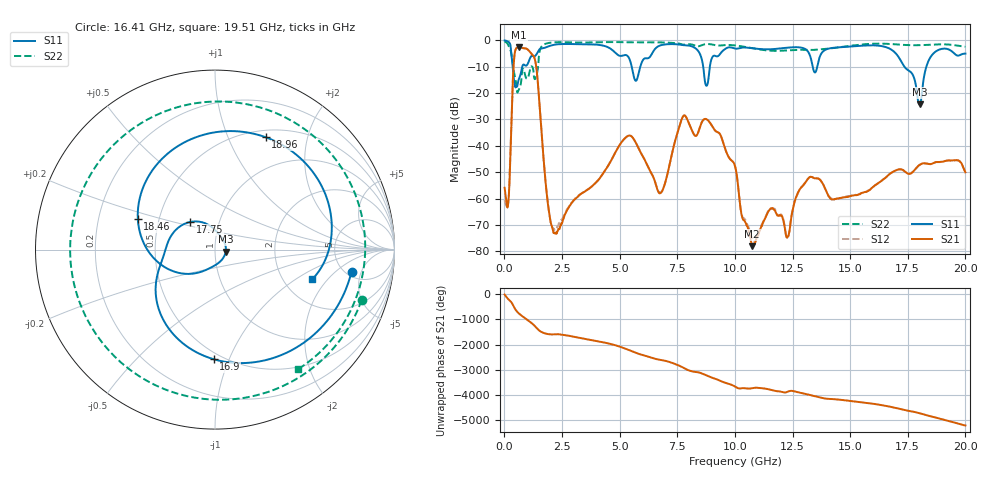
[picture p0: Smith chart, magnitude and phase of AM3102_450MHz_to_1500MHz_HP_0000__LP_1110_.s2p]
!Agilent Technologies,E8364B,MY43040894,A.07.50.67
!Agilent E8364B: A.07.50.67
!Date: Thursday, January 11, 2018 05:18:35
!Correction: S11(Full 2 Port(1,2))
!S21(Full 2 Port(1,2))
!S12(Full 2 Port(1,2))
!S22(Full 2 Port(1,2))
!S2P File: Measurements: S11, S21, S12, S22:
# Hz S  dB  R 50
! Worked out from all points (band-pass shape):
!   1601 points, 10 MHz to 20 GHz, reference 50 ohm
!   highest |S21| = -2.59 dB at 634.7 MHz (marker M1); lowest = -78.1 dB at 10.75 GHz (marker M2)
!   |S21| within 3 dB of the highest: 439 MHz to 1.232 GHz (792.8 MHz wide, 94.9 % of centre)
!   lowest |S11| = -24.3 dB at 18.01 GHz (marker M3), VSWR 1.13, Z = 56.3 - j1.3 ohm
!   |S11| at or under -10 dB: 358.5 MHz to 774.2 MHz (415.6 MHz wide, 73.4 % of centre); 5.524 GHz to 5.897 GHz (373.3 MHz wide, 6.54 % of centre); 17.36 GHz to 18.31 GHz (950.9 MHz wide, 5.33 % of centre)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
!   |S22| runs from -19.8 to -0.5 dB; largest |S21 - S12| = 0.0019
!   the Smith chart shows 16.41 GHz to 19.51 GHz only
!   S11 on the Smith chart (normalised r, x): 16.41 GHz: 5.62, -3.39; 16.9 GHz: 0.45, -0.88; 17.75 GHz: 0.73, +0.23; 18.46 GHz: 0.38, +0.16; 18.96 GHz: 0.58, +1.38; 19.51 GHz: 2.85, -1.39
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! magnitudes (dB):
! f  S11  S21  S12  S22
! 10 MHz  -0.1  -55.9  -60.7  -0.5
! 172.4 MHz  -0.6  -61.3  -61.2  -1.9
! 422.3 MHz  -15.4  -7.0  -7.0  -12.3
! 634.7 MHz  -14.6  -2.6  -2.6  -18.6
! 1.347 GHz  -5.8  -8.1  -8.1  -14.5
! 2.109 GHz  -1.8  -72.3  -71.3  -0.8
! 3.346 GHz  -1.5  -58.1  -58.1  -0.8
! 5.42 GHz  -7.0  -36.1  -36.1  -0.7
! 6.682 GHz  -2.2  -57.5  -57.3  -0.8
! 7.794 GHz  -1.8  -28.5  -28.5  -1.7
! 10.01 GHz  -3.1  -47.7  -47.6  -1.9
! 10.75 GHz  -3.0  -78.1  -74.9  -3.0
! 13.34 GHz  -8.5  -51.8  -51.9  -3.6
! 16.41 GHz  -2.3  -52.9  -52.8  -1.3
! 16.68 GHz  -3.0  -51.0  -50.9  -1.4
! 16.9 GHz  -4.3  -49.7  -49.7  -1.5
! 17.75 GHz  -13.7  -49.6  -49.7  -1.9
! 18.01 GHz  -24.3  -47.3  -47.2  -1.8
! 18.46 GHz  -6.7  -46.9  -47.0  -1.7
! 18.96 GHz  -3.3  -46.1  -46.1  -1.5
! 19.51 GHz  -4.9  -45.5  -45.5  -1.8
! 20 GHz  -5.0  -50.1  -49.9  -2.4
